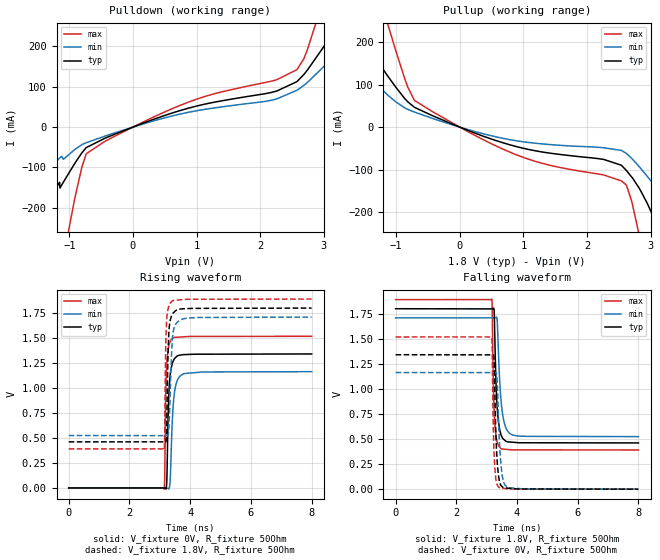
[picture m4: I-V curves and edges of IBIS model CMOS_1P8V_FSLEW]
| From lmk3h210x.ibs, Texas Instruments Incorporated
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[Model]   CMOS_1P8V_FSLEW
Model_type   Output
Polarity   Non-Inverting
Vmeas = 0.9
Vref = 0.9
Cref = 2pF
Rref = 100000
|   typ   min   max
C_comp   2.5pF   2pF   3pF
[Voltage Range]   1.8   1.71   1.89
[Temperature Range]   45   125   -40
[Pullup Reference]   1.8   1.71   1.89
[Pulldown Reference]   -0   0   -0
[Power Clamp Reference]   1.8   1.71   1.89
[GND Clamp Reference]   0   0   0
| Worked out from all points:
|   slope of the pulldown table from 0 to 0.27 V, typ, clamps not added: 16.7 ohm
|   slope of the pullup table from 0 to 0.27 V, typ, clamps not added: 17 ohm
|   falling waveform, V_fixture 1.8V, R_fixture 50Ohm: 20-80 % time 102ps typ, 143ps min, 69.6ps max; typ from 1.8 V to 0.461 V
|   rising waveform, V_fixture 0V, R_fixture 50Ohm: 20-80 % time 79.2ps typ, 112ps min, 55.2ps max; typ from 0.001 V to 1.34 V
|   rising waveform, V_fixture 1.8V, R_fixture 50Ohm: 20-80 % time 62ps typ, 88.8ps min, 45.3ps max; typ from 0.461 V to 1.8 V
|   falling waveform, V_fixture 0V, R_fixture 50Ohm: 20-80 % time 85.4ps typ, 110ps min, 61.9ps max; typ from 1.34 V to 0 V
[Pulldown]
|   Voltage   I(typ)   I(min)   I(max)
-1.8V     -365.8mA   -207.1mA   -1.065A
-1.249V   -164.3mA   -92.85mA   -468.1mA
-1.12V    -143.7mA   -72.05mA   -359.7mA
-1.033V   -120.9mA   -71.78mA   -275.7mA
-801mV    -63.48mA   -43.35mA   -98.65mA
-730.8mV  -50.55mA   -38.44mA   -65.82mA
802.8mV   43.86mA    34.47mA    57.71mA
2.266V    89.82mA    70.29mA    117.9mA
2.579V    112.9mA    91.44mA    142.5mA
2.741V    141.1mA    110.5mA    191.7mA
3.065V    214mA      160.1mA    349.7mA
3.6V      343.6mA    250.7mA    637.5mA
[Pullup]
|   Voltage   I(typ)   I(min)   I(max)
-1.8V     266.6mA    175.5mA    585.6mA
-1.136V   121.3mA    76.01mA    244.8mA
-822.6mV  60.6mA     42.27mA    96.52mA
-709.2mV  46.52mA    35.37mA    62.81mA
235.8mV   -13.89mA   -10.25mA   -19.26mA
900mV     -46.21mA   -32.39mA   -65.71mA
2.266V    -76.3mA    -48.77mA   -112.9mA
2.547V    -90.95mA   -55.37mA   -127.3mA
2.623V    -102.7mA   -62.57mA   -138mA
2.817V    -143.1mA   -92.52mA   -252.4mA
3.136V    -244.5mA   -152.2mA   -549.1mA
3.6V      -420.8mA   -256.8mA   -1.061A
[Ramp]
R_load = 50
|   typ   min   max
dV/dt_r   0.803846/7.87714e-11   0.697158/1.10948e-10   0.909961/5.4711e-11
dV/dt_f   0.802494/1.01447e-10   0.710091/1.42757e-10   0.89905/6.95359e-11
[Falling Waveform]
V_fixture = 1.8V
V_fixture_min = 1.71V
V_fixture_max = 1.89V
R_fixture = 50Ohm
C_fixture = 0F
|   Time   V(typ)   V(min)   V(max)
0s        1.798V     1.707V     1.889V
3.168ns   1.797V     1.707V     1.895V
3.182ns   1.797V     1.707V     1.819V
3.224ns   1.803V     1.707V     1.005V
3.262ns   1.609V     1.707V     688.8mV
3.343ns   833.2mV    1.691V     474.1mV
3.468ns   547.2mV    906.2mV    405.6mV
3.613ns   482.7mV    626.3mV    397.7mV
3.858ns   467.7mV    540.2mV    391.6mV
8ns       460.8mV    523.8mV    390.6mV
[Rising Waveform]
V_fixture = 0V
V_fixture_min = 0V
V_fixture_max = 0V
R_fixture = 50Ohm
C_fixture = 0F
|   Time   V(typ)   V(min)   V(max)
0s        686uV      1.304mV    346.6uV
3.143ns   681.2uV    748.4uV    -11.78mV
3.162ns   -706.2uV   745uV      99.05mV
3.197ns   -8.485mV   738.8uV    937.6mV
3.23ns    60.86mV    -1.415mV   1.242V
3.303ns   962.9mV    -7.421mV   1.428V
3.345ns   1.137V     89.89mV    1.467V
3.44ns    1.267V     814mV      1.502V
3.807ns   1.334V     1.144V     1.512V
8ns       1.34V      1.163V     1.517V
[Rising Waveform]
V_fixture = 1.8V
V_fixture_min = 1.71V
V_fixture_max = 1.89V
R_fixture = 50Ohm
C_fixture = 0F
|   Time   V(typ)   V(min)   V(max)
0s        461.3mV    524.7mV    390.8mV
3.143ns   461.5mV    523.3mV    380.2mV
3.161ns   459.9mV    523.3mV    505.6mV
3.195ns   455.1mV    523.3mV    1.387V
3.226ns   601.2mV    523.3mV    1.673V
3.264ns   1.241V     524.2mV    1.776V
3.299ns   1.552V     602.3mV    1.819V
3.414ns   1.735V     1.483V     1.872V
3.915ns   1.794V     1.699V     1.887V
8ns       1.799V     1.709V     1.889V
[Falling Waveform]
|Gnd
V_fixture = 0V
V_fixture_min = 0V
V_fixture_max = 0V
R_fixture = 50Ohm
C_fixture = 0F
|   Time   V(typ)   V(min)   V(max)
0s        1.34V      1.162V     1.517V
3.165ns   1.339V     1.162V     1.517V
3.182ns   1.338V     1.162V     1.42V
3.22ns    1.338V     1.162V     604.9mV
3.254ns   1.219V     1.162V     297.1mV
3.32ns    427mV      1.154V     69.16mV
3.414ns   90.9mV     515mV      15.55mV
3.515ns   23.78mV    132.8mV    9.126mV
3.72ns    9.496mV    14.93mV    2.869mV
8ns       159.8uV    308.1uV    72.42uV
